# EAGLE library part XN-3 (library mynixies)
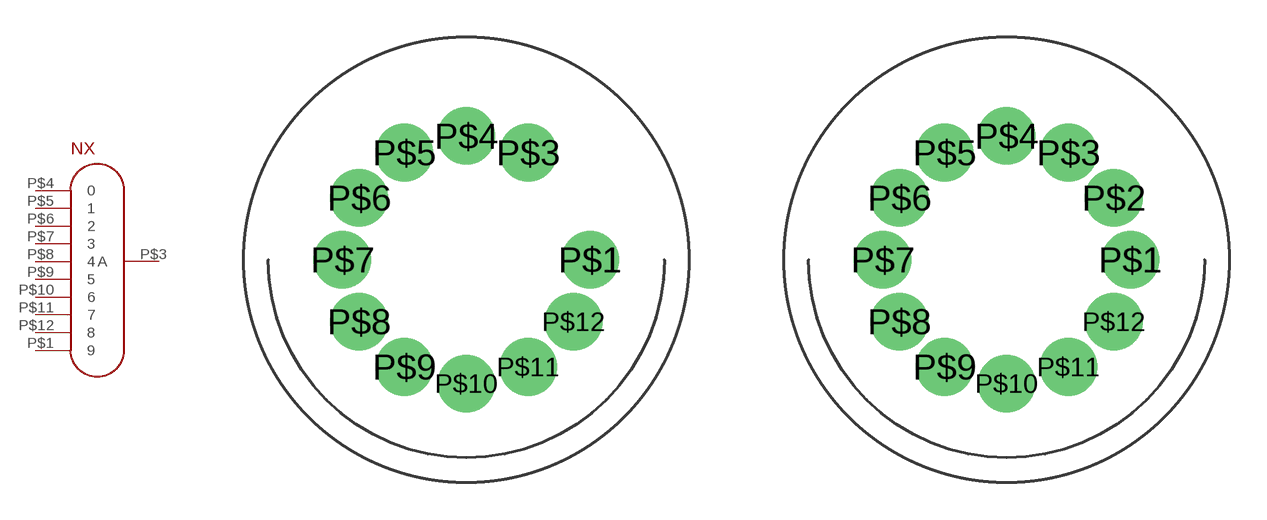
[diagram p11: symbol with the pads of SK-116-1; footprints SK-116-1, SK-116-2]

Designator prefix NX

## XN-3  [SK-116-1]
P$1  9
P$3  A
P$4  0
P$5  1
P$6  2
P$7  3
P$8  4
P$9  5
P$10  6
P$11  7
P$12  8

## XN-3XN-12  [SK-116-2]
P$1  9
P$2  0
P$3  A
P$5  1
P$6  2
P$7  3
P$8  4
P$9  5
P$10  6
P$11  7
P$12  8

## Footprint SK-116-1 (pad centres in mm)
drill 1.55: P$1 5,0; P$3 2.5,4.33; P$4 0,5; P$5 -2.5,4.33; P$6 -4.33,2.5; P$7 -5,0; P$8 -4.33,-2.5; P$9 -2.5,-4.33; P$10 0,-5; P$11 2.5,-4.33; P$12 4.33,-2.5

## Footprint SK-116-2 (pad centres in mm)
drill 1.55: P$1 5,0; P$2 4.33,2.5; P$3 2.5,4.33; P$4 0,5; P$5 -2.5,4.33; P$6 -4.33,2.5; P$7 -5,0; P$8 -4.33,-2.5; P$9 -2.5,-4.33; P$10 0,-5; P$11 2.5,-4.33; P$12 4.33,-2.5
